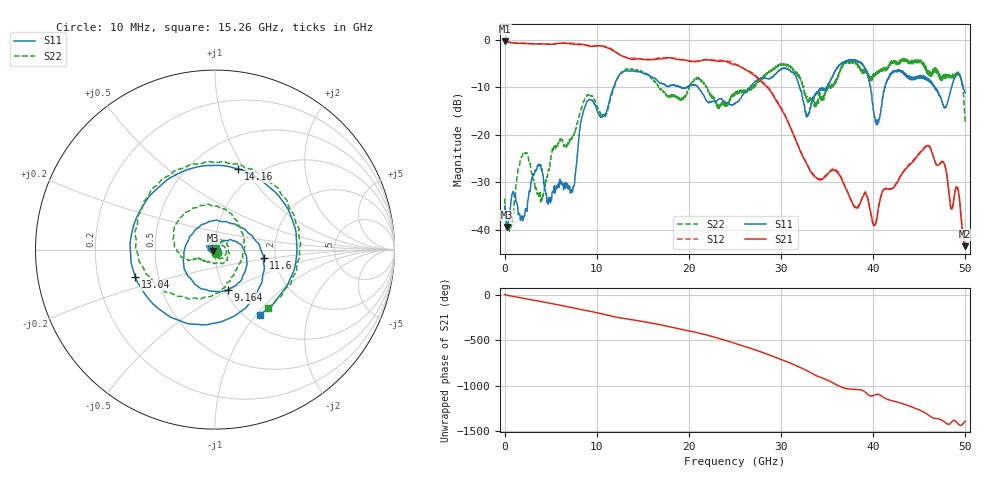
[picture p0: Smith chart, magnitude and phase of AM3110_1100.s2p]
# Hz S DB R 50.0
!freq dBS11 angS11 dBS21 angS21 dBS12 angS12 dBS22 angS22
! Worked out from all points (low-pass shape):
!   1601 points, 10 MHz to 50 GHz, reference 50 ohm
!   highest |S21| = -0.18 dB at 10 MHz (marker M1); lowest = -43.5 dB at 49.94 GHz (marker M2)
!   |S21| within 3 dB of the highest: start of sweep to 12.52 GHz
!   lowest |S11| = -39.5 dB at 291.2 MHz (marker M3), VSWR 1.02, Z = 49.1 - j0.526 ohm
!   |S11| at or under -10 dB: start of sweep to 11.82 GHz; 21.01 GHz to 26.61 GHz (5.604 GHz wide, 23.5 % of centre); 32 GHz to 34.95 GHz (2.947 GHz wide, 8.8 % of centre)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
!   |S22| runs from -40.4 to -3.8 dB; largest |S21 - S12| = 0.026
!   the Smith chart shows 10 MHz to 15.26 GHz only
!   S11 on the Smith chart (normalised r, x): 10 MHz: 1.02, -0.03; 9.164 GHz: 1.04, -0.49; 11.6 GHz: 1.73, -0.17; 13.04 GHz: 0.37, -0.15; 14.16 GHz: 0.82, +0.94; 15.26 GHz: 1.16, -1.05
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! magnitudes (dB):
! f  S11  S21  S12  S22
! 10 MHz  -35.0  -0.2  -0.1  -33.5
! 291.2 MHz  -39.5  -0.4  -0.3  -39.0
! 1.978 GHz  -38.2  -0.7  -0.6  -24.1
! 3.947 GHz  -26.5  -0.8  -0.8  -33.7
! 7.352 GHz  -32.1  -0.8  -0.7  -20.4
! 8.352 GHz  -16.5  -0.9  -0.9  -14.2
! 9.164 GHz  -12.6  -1.3  -1.1  -11.6
! 11.6 GHz  -11.2  -2.0  -1.9  -11.7
! 13.04 GHz  -6.6  -3.6  -3.6  -6.2
! 14.16 GHz  -6.6  -4.0  -3.8  -6.3
! 15.26 GHz  -7.1  -4.1  -4.0  -7.1
! 16.69 GHz  -8.8  -4.0  -3.8  -9.8
! 25 GHz  -13.4  -5.2  -5.0  -11.4
! 30.38 GHz  -5.9  -15.8  -15.6  -5.0
! 33.35 GHz  -13.2  -28.2  -27.9  -12.9
! 38.13 GHz  -4.2  -35.4  -35.5  -4.6
! 40.47 GHz  -17.8  -36.7  -36.6  -7.0
! 41.69 GHz  -7.9  -31.4  -31.4  -5.9
! 46 GHz  -8.2  -22.3  -22.2  -6.7
! 49.16 GHz  -7.2  -31.3  -31.1  -7.5
! 49.94 GHz  -11.0  -43.5  -42.8  -15.6
! 50 GHz  -11.1  -43.4  -42.7  -17.7
